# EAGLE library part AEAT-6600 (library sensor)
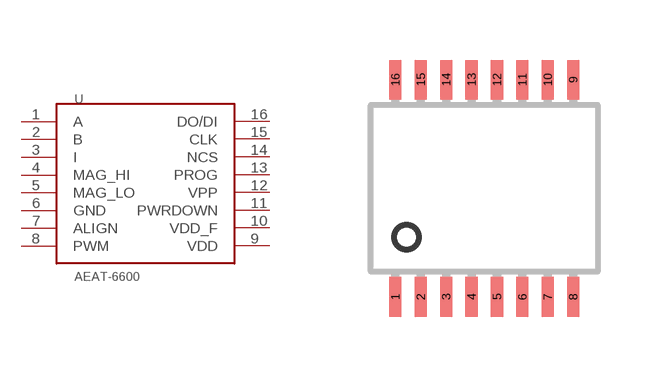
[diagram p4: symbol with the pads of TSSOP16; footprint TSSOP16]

Designator prefix U

## AEAT-6600  [TSSOP16]
1  A
2  B
3  I
4  MAG_HI
5  MAG_LO
6  GND
7  ALIGN
8  PWM
9  VDD
10  VDD_F
11  PWRDOWN
12  VPP
13  PROG
14  NCS
15  CLK
16  DO/DI

## Footprint TSSOP16 (pad centres in mm)
Thin Shrink Small Outline Plastic 14
smd 0.305 x 0.991: 1 -2.53,-2.718; 2 -1.895,-2.718; 3 -1.26,-2.718; 4 -0.625,-2.718; 5 0.01,-2.718; 6 0.645,-2.718; 7 1.28,-2.718; 8 1.915,-2.718; 9 1.915,2.718; 10 1.28,2.718; 11 0.645,2.718; 12 0.01,2.718; 13 -0.625,2.718; 14 -1.26,2.718; 15 -1.895,2.718; 16 -2.53,2.718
